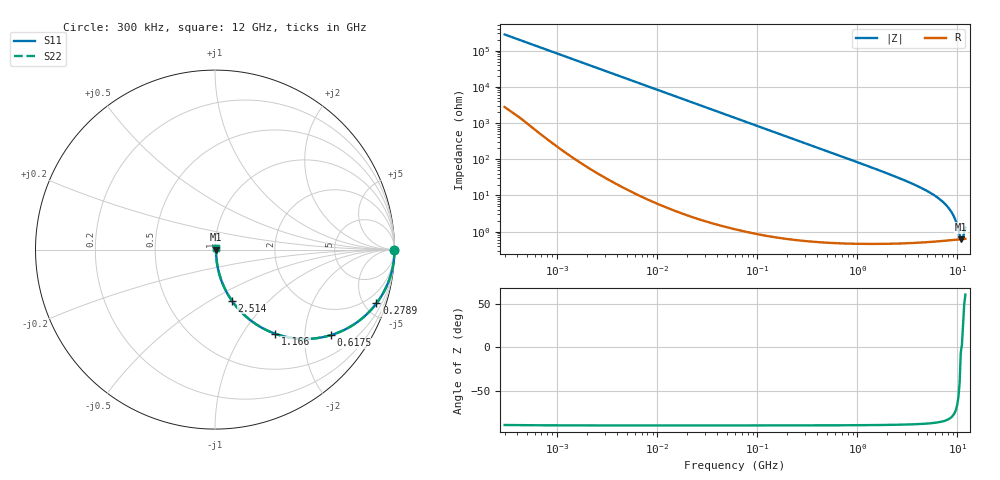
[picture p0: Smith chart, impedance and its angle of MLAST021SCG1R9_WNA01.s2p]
! MLAST021SCG1R9_WNA01  S-PARAMETER MODEL  ( General Type )
! Model Generated by TAIYO YUDEN Corporation (http://www.ty-top.com)
! Version 1.0
! TAIYO YUDEN Control No. 220901
! Copyright(c) 2022 TAIYO YUDEN CO.,LTD. All Rights Reserved.
! Product Description (link to TY-COMPAS)
! https://ds.yuden.co.jp/TYCOMPAS/or/detail?pn=MLAST021SCG1R9BWNA01&u=M
! Products Name : Multilayer Ceramic Capacitors
! Characteristics :
!  Capacitance : 1.9 pF , Rated Voltage : 25V , TCC : CG / C0G
!  Case Size : 0.25 x 0.125 / 0.0098 x 0.0049 [mm/inch] , Thickness : 0.125 / 0.0049 [mm/inch]
!  (Conditions: Temperature = 25 degC , DC Bias Current/Voltage = 0A / 0V)
! External Node Assignments :
!  1  o---| |---o  2
! GND o---------o GND
! Frequency Range : 0.3MHz  -  12000MHz  [ 401 STEP ]
# MHz S RI R 50
! Freq[MHz].  S11 Real  S11 Imag  S21 Real  S21 Imag  S12 Real  S12 Imag  S22 Real  S22 Imag
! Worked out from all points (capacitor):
!   401 points, 300 kHz to 12 GHz, reference 50 ohm
!   read as one part in series: C = 1.9 pF near 316.3 kHz
!   lowest |Z| = 620 mohm at 10.79 GHz (marker M1)
!   series resonance near 10.98 GHz, so ESL is about 110 pH
!   S11 on the Smith chart (normalised r, x): 300 kHz: open; 278.9 MHz: 1.01, -6.00; 617.5 MHz: 1.01, -2.70; 1.166 GHz: 1.01, -1.42; 2.514 GHz: 1.01, -0.63; 12 GHz: 1.01, +0.02
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0.3  1 -0.000358  3.69e-06 0.000358  3.69e-06 0.000358  1 -0.000358
1.769972  1 -0.00211  7.84e-06 0.00211  7.84e-06 0.00211  1 -0.00211
10.44266  0.9998 -0.0125  0.000164 0.0125  0.000164 0.0125  0.9998 -0.0125
60  0.9948 -0.0713  0.00516 0.0713  0.00516 0.0713  0.9948 -0.0713
132.8329  0.9753 -0.1547  0.0247 0.1547  0.0247 0.1547  0.9753 -0.1547
278.9009  0.8996 -0.2995  0.1004 0.2995  0.1004 0.2995  0.8996 -0.2995
353.9943  0.8476 -0.3583  0.1524 0.3583  0.1524 0.3583  0.8476 -0.3583
617.4538  0.646 -0.4764  0.354 0.4764  0.354 0.4764  0.646 -0.4764
848.5281  0.4905 -0.4975  0.5095 0.4975  0.5095 0.4975  0.4905 -0.4975
1166.079  0.3362 -0.4692  0.6638 0.4692  0.6638 0.4692  0.3362 -0.4692
2088.533  0.1328 -0.3334  0.8672 0.3334  0.8672 0.3334  0.1328 -0.3334
2514.07  0.0939 -0.2844  0.9061 0.2844  0.9061 0.2844  0.0939 -0.2844
4875.354  0.0233 -0.1334  0.9767 0.1334  0.9767 0.1334  0.0233 -0.1334
6026.253  0.0144 -0.0944  0.9856 0.0944  0.9856 0.0944  0.0144 -0.0944
7254.098  0.00956 -0.0631  0.9904 0.0631  0.9904 0.0631  0.00956 -0.0631
8064.993  0.00783 -0.0461  0.9922 0.0461  0.9922 0.0461  0.00783 -0.0461
8966.534  0.00672 -0.0295  0.9933 0.0295  0.9933 0.0295  0.00672 -0.0295
9454.42  0.00638 -0.0213  0.9936 0.0213  0.9936 0.0213  0.00638 -0.0213
10511.28  0.00612 -0.0052  0.9939 0.0052  0.9939 0.0052  0.00612 -0.0052
10793.46  0.00614 -0.00062  0.9939 0.00062  0.9939 0.00062  0.00614 -0.00062
11083.22  0.00617 0.000327  0.9938 -0.000327  0.9938 -0.000327  0.00617 0.000327
12000  0.00643 0.0112  0.9936 -0.0112  0.9936 -0.0112  0.00643 0.0112
